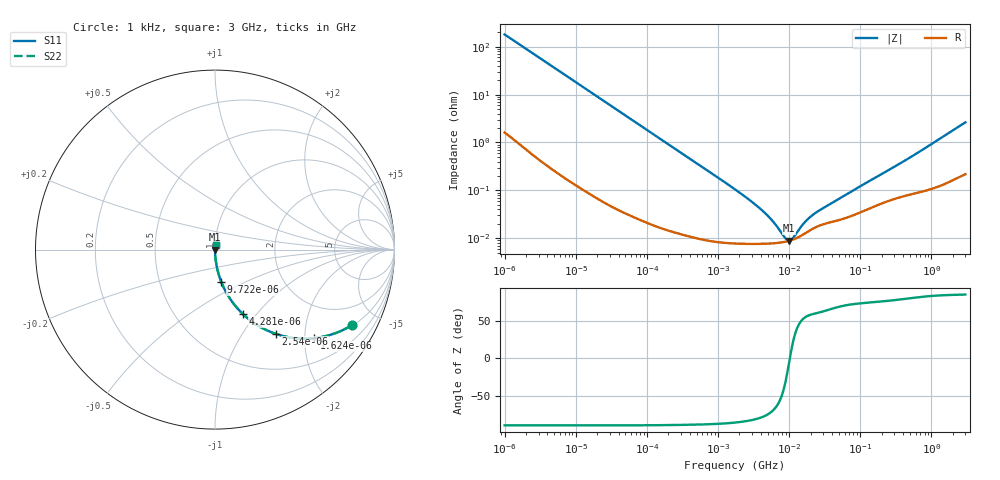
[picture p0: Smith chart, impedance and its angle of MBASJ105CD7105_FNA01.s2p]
! MBASJ105CD7105_FNA01  S-PARAMETER MODEL  ( Standard Model )
! Model Generated by TAIYO YUDEN Corporation (http://www.ty-top.com)
! Version 1.0
! TAIYO YUDEN Control No. 220601
! Copyright(c) 2020 TAIYO YUDEN CO.,LTD. All Rights Reserved.
! Product Description (link to TY-COMPAS)
! https://ds.yuden.co.jp/TYCOMPAS/or/detail?pn=MBASJ105CD7105KFNA01&u=M
! Products Name : Multilayer Ceramic Capacitors
! Characteristics :
!  Capacitance : 1 [uF] , Rated Voltage : 6.3 [V] , TCC : X7T
!  Case Size : 1.0 x 0.5 / 0.039 x 0.02 [mm/inch] , Thickness : 0.5 / 0.02 [mm/inch]
!  (Conditions: Temperature = 25 [degC] , DC Bias Voltage = 0 [V])
! External Node Assignments :
!  1  o---| |---o  2
! GND o---------o GND
! Frequency Range : 1kHz  -  3GHz  [ 401 STEP ]
# MHZ S RI R 50
! Freq[MHz].  S11 Real  S11 Imag  S21 Real  S21 Imag  S12 Real  S12 Imag  S22 Real  S22 Imag
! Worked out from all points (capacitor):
!   401 points, 1 kHz to 3 GHz, reference 50 ohm
!   read as one part in series: C = 880 nF near 1.077 kHz
!   lowest |Z| = 8.87 mohm at 9.991 MHz (marker M1)
!   series resonance near 10.22 MHz, so ESL is about 280 pH
!   S11 on the Smith chart (normalised r, x): 1 kHz: 1.03, -3.61; 1.624 kHz: 1.02, -2.23; 2.54 kHz: 1.01, -1.43; 4.281 kHz: 1.01, -0.85; 9.722 kHz: 1.00, -0.38; 3 GHz: 1.00, +0.05
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0.001  0.7631 -0.4208  0.2369 0.4208  0.2369 0.4208  0.7631 -0.4208
0.001624  0.5537 -0.493  0.4463 0.493  0.4463 0.493  0.5537 -0.493
0.00254  0.3389 -0.4696  0.6611 0.4696  0.6611 0.4696  0.3389 -0.4696
0.004281  0.1545 -0.358  0.8455 0.358  0.8455 0.358  0.1545 -0.358
0.006215  0.0806 -0.2688  0.9194 0.2688  0.9194 0.2688  0.0806 -0.2688
0.009722  0.0352 -0.1807  0.9648 0.1807  0.9648 0.1807  0.0352 -0.1807
0.01216  0.023 -0.1465  0.977 0.1465  0.977 0.1465  0.023 -0.1465
0.033275  0.00346 -0.0549  0.9965 0.0549  0.9965 0.0549  0.00346 -0.0549
0.147855  0.000323 -0.0125  0.9997 0.0125  0.9997 0.0125  0.000323 -0.0125
1.732051  7.85e-05 -0.00105  0.9999 0.00105  0.9999 0.00105  7.85e-05 -0.00105
2.919173  7.63e-05 -0.000588  0.9999 0.000588  0.9999 0.000588  7.63e-05 -0.000588
4.238263  7.66e-05 -0.000366  0.9999 0.000366  0.9999 0.000366  7.66e-05 -0.000366
5.928204  7.83e-05 -0.00021  0.9999 0.00021  0.9999 0.00021  7.83e-05 -0.00021
8.606987  8.38e-05 -6.32e-05  0.9999 6.32e-05  0.9999 6.32e-05  8.38e-05 -6.32e-05
9.991309  8.83e-05 -8.06e-06  0.9999 8.06e-06  0.9999 8.06e-06  8.83e-05 -8.06e-06
11.59828  9.51e-05 4.65e-05  0.9999 -4.65e-05  0.9999 -4.65e-05  9.51e-05 4.65e-05
16.22291  0.000123 0.000168  0.9999 -0.000168  0.9999 -0.000168  0.000123 0.000168
21.06097  0.000155 0.000257  0.9998 -0.000257  0.9998 -0.000257  0.000155 0.000257
29.45871  0.000193 0.00037  0.9998 -0.00037  0.9998 -0.00037  0.000193 0.00037
256.0921  0.000615 0.00264  0.9994 -0.00264  0.9994 -0.00264  0.000615 0.00264
581.6181  0.000891 0.00549  0.9991 -0.00549  0.9991 -0.00549  0.000891 0.00549
3000  0.00286 0.0261  0.9971 -0.0261  0.9971 -0.0261  0.00286 0.0261
